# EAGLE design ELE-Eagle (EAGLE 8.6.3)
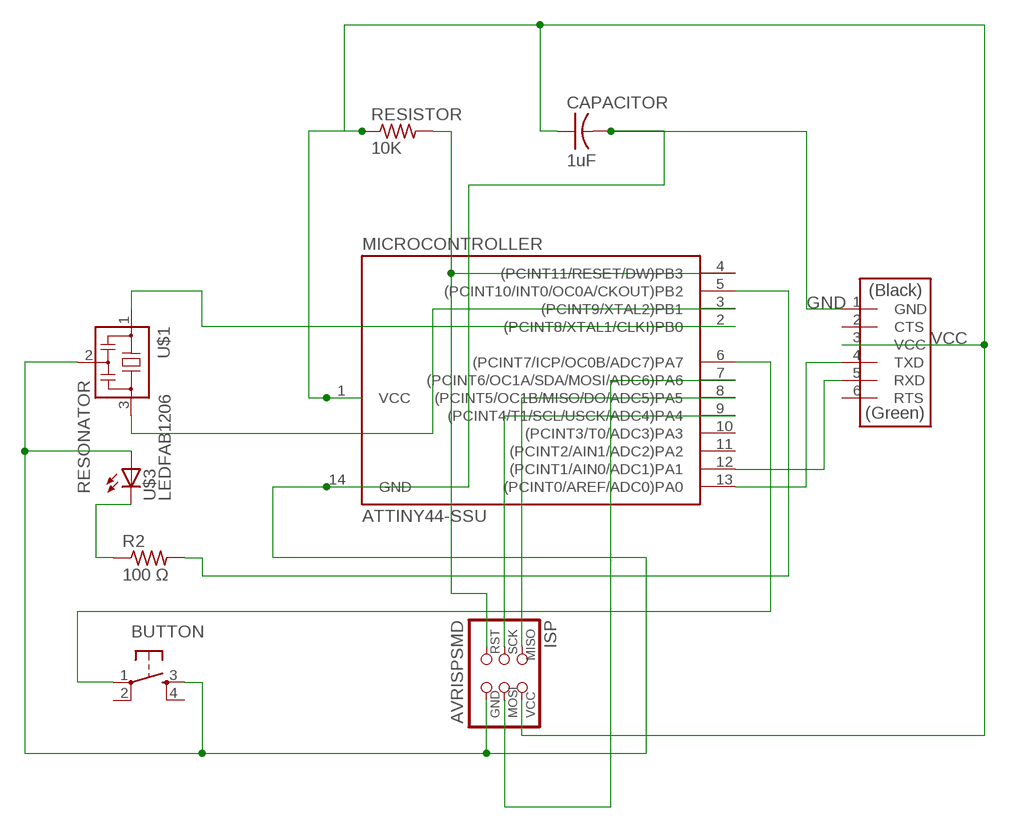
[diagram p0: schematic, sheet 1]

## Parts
BUTTON  6MM_SWITCH6MM_SWITCH  [6MM_SWITCH]
CAPACITOR  1uF  CAP-US1206FAB  [C1206FAB]
ISP  AVRISPSMD  [2X03SMD]
MICROCONTROLLER  ATTINY44-SSU  [SOIC14]
R2  100 Ω  RES-US1206FAB  [R1206FAB]
RESISTOR  10K  RES-US1206FAB  [R1206FAB]
U$1  RESONATOR  [EFOBM]
U$2  FTDI-SMD-HEADER  [1X06SMD]
U$3  LEDFAB1206  [LED1206FAB]

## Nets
GND: BUTTON.3(S) CAPACITOR.2 ISP.6(GND) MICROCONTROLLER.14(GND) U$1.2 U$2.1(GND) U$3.1(A)
N$1: BUTTON.1(P) MICROCONTROLLER.6((PCINT7/ICP/OC0B/ADC7)PA7)
N$2: ISP.4(MOSI) MICROCONTROLLER.7((PCINT6/OC1A/SDA/MOSI/ADC6)PA6)
N$4: MICROCONTROLLER.2((PCINT8/XTAL1/CLKI)PB0) U$1.1
N$5: MICROCONTROLLER.3((PCINT9/XTAL2)PB1) U$1.3
N$8: MICROCONTROLLER.13((PCINT0/AREF/ADC0)PA0) U$2.4(TXD)
N$9: MICROCONTROLLER.12((PCINT1/AIN0/ADC1)PA1) U$2.5(RXD)
N$10: ISP.5(RST) MICROCONTROLLER.4((PCINT11/RESET/DW)PB3) RESISTOR.2
N$11: ISP.3(SCK) MICROCONTROLLER.9((PCINT4/T1/SCL/USCK/ADC4)PA4)
N$12: ISP.1(MISO) MICROCONTROLLER.8((PCINT5/OC1B/MISO/DO/ADC5)PA5)
N$13: MICROCONTROLLER.5((PCINT10/INT0/OC0A/CKOUT)PB2) R2.2
N$14: R2.1 U$3.2(C)
VCC: CAPACITOR.1 ISP.2(VCC) MICROCONTROLLER.1(VCC) RESISTOR.1 U$2.3(VCC)
Unconnected: BUTTON.2(P1) BUTTON.4(S1) MICROCONTROLLER.10((PCINT3/T0/ADC3)PA3) MICROCONTROLLER.11((PCINT2/AIN1/ADC2)PA2) U$2.2(CTS) U$2.6(RTS)

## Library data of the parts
BUTTON = fab:6MM_SWITCH: OMRON SWITCH
CAPACITOR = fab:CAP-US
ISP = fab:AVRISP
MICROCONTROLLER = fab:ATTINY44
R2 RESISTOR = fab:RES-US: Resistor (US Symbol)
U$1 = fab:RESONATOR
U$2 = fab:FTDI-SMD-HEADER
U$3 = fab:LED: LED

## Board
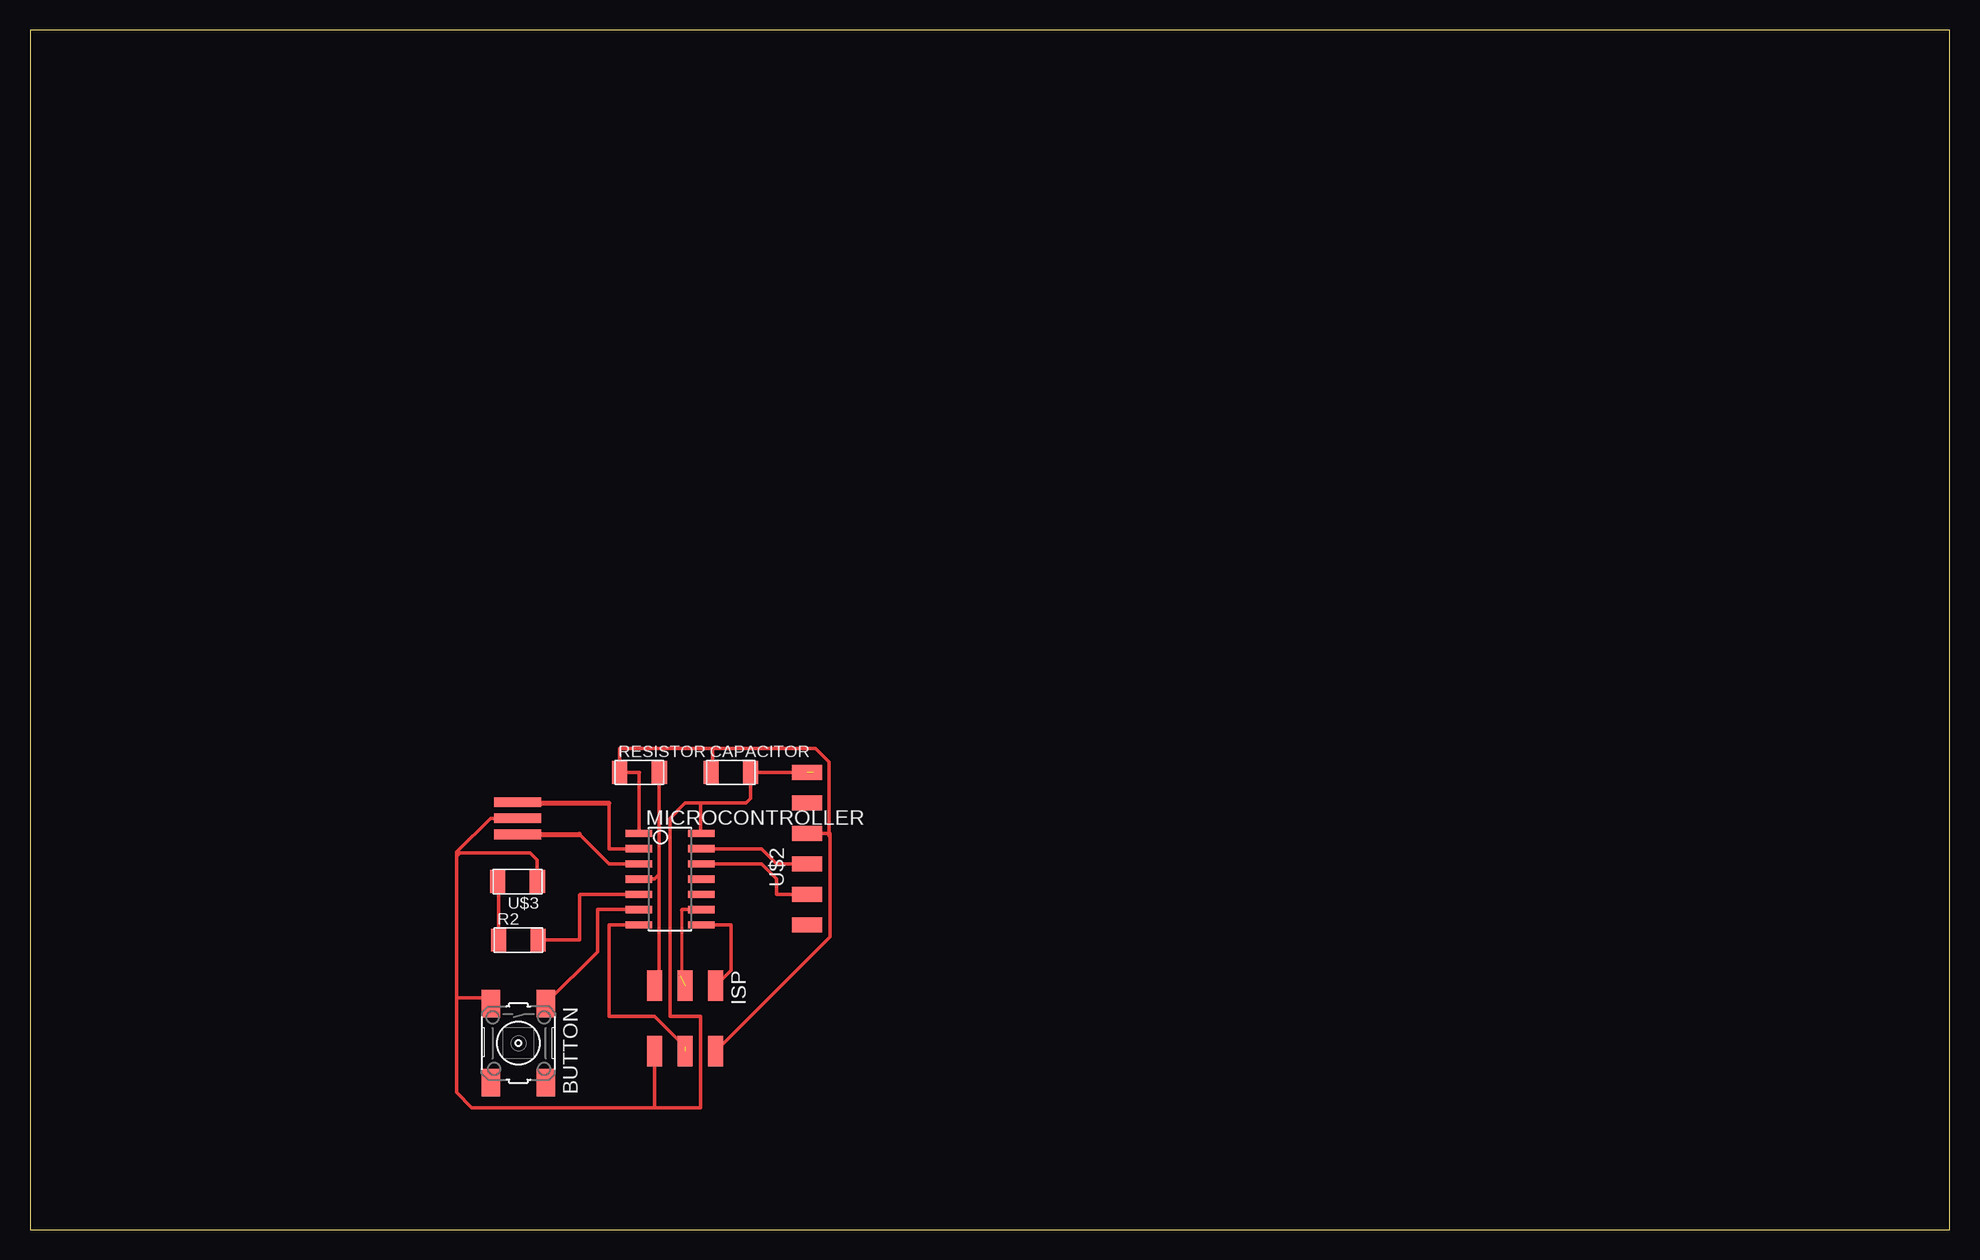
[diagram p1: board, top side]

Size 160 x 100 mm. Coordinates in mm from the lower left corner, seen from the top.
Outline: 0,0 160,0 160,100 0,100 0,0
Copper layers (1*16): Top 0.035mm / dielectric 1.5mm / Bottom 0.035mm
Design rules "default *": minimum track width 12mil, minimum drill 24mm, track to track 16mil, track to pad 16mil, pad to pad 16mil, via to via 16mil, smd to smd 6mil, copper to edge 40mil, drill to drill 6mil, minimum pad ring 10mil, minimum via ring 8mil, stop-mask expansion 4mil, vias tented up to drill 0mil, thermal gap 10mil

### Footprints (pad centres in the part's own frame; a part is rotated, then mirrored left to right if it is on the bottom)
6MM_SWITCH = smd 2.286 x 1.524: 1 -3.302,2.286; 2 3.302,2.286; 3 -3.302,-2.286; 4 3.302,-2.286
C1206FAB = smd 1.27 x 1.905: 1 -1.651,0; 2 1.651,0
2X03SMD = smd 2.54 x 1.27: 1 -2.54,2.54; 2 2.92,2.54; 3 -2.54,0; 4 2.92,0; 5 -2.54,-2.54; 6 2.92,-2.54
SOIC14 = smd 0.61 x 2.21: 1 -3.81,-2.603; 2 -2.54,-2.603; 3 -1.27,-2.603; 4 0,-2.603; 5 1.27,-2.603; 6 2.54,-2.603; 7 3.81,-2.603; 8 3.81,2.603; 9 2.54,2.603; 10 1.27,2.603; 11 0,2.603; 12 -1.27,2.603; 13 -2.54,2.603; 14 -3.81,2.603
R1206FAB = smd 1.27 x 1.905: 1 -1.651,0; 2 1.651,0
EFOBM = smd 0.8 x 3.9: 1 -1.35,0; 2 0,0; 3 1.35,0
1X06SMD = smd 2.54 x 1.27: 1 0,6.35; 2 0,3.81; 3 0,1.27; 4 0,-1.27; 5 0,-3.81; 6 0,-6.35
LED1206FAB = smd 1.27 x 1.905: 1 -1.651,0; 2 1.651,0

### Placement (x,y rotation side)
BUTTON  40.71,15.54 270 top
CAPACITOR  58.42,38.1 0 top
ISP  54.61,17.78 270 top
MICROCONTROLLER  53.34,29.21 270 top
R2  40.71,24.13 0 top
RESISTOR  50.8,38.1 0 top
U$1  40.64,34.29 270 top
U$2  64.77,31.75 0 top
U$3  40.64,29.01 180 top

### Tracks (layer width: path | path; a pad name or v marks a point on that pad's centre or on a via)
GND  (1 unrouted)
  Top 0.152: MICROCONTROLLER.14 55.88,33.08
  Top 0.305: U$1.2 38.39,34.29 35.56,31.46 35.56,31.1 | 35.56,31.1 35.56,19.3 | 35.56,19.3 35.56,11.43 36.83,10.16 52.07,10.16 | 52.07,10.16 ISP.6 | 52.07,10.16 55.88,10.16 55.88,17.78 53.34,17.78 53.34,34.29 54.61,35.56 55.88,35.56 | 55.88,35.56 59.69,35.56 60.07,35.94 CAPACITOR.2 65.3,38.1 | 55.88,33.08 55.88,35.56 | BUTTON.3 37.97,19.3 35.56,19.3 | U$3.1 42.29,30.81 41.7,31.4 35.86,31.4 35.56,31.1
N$1
  Top 0.305: BUTTON.1 47.3,23.15 47.3,26.7 50.71,26.7 MICROCONTROLLER.6
N$2  (1 unrouted)
  Top 0.305: MICROCONTROLLER.7 48.26,25.4 48.26,17.78 52.07,17.78 54.61,15.24
N$4
  Top 0.152: U$1.1 40.72,35.56
  Top 0.305: 48.26,35.56 48.26,31.75 MICROCONTROLLER.2
  Top 0.406: 40.72,35.56 48.26,35.56
N$5
  Top 0.305: 45.8,32.94 48.26,30.48 MICROCONTROLLER.3
  Top 0.406: U$1.3 45.8,32.94
N$8
  Top 0.305: MICROCONTROLLER.13 60.96,31.75 62.23,30.48 U$2.4
N$9
  Top 0.305: MICROCONTROLLER.12 60.96,30.48 62.23,29.21 62.23,27.94 U$2.5
N$10
  Top 0.152: 52.45,20.7 ISP.5
  Top 0.305: RESISTOR.2 52.45,29.59 | 52.45,29.59 52.07,29.21 MICROCONTROLLER.4 | 52.45,29.59 52.45,20.7
N$11  (1 unrouted)
  Top 0.254: 54.3,26.6 54.3,21.3
  Top 0.305: MICROCONTROLLER.9 54.37,26.67 54.3,26.6 | 54.3,21.3 54.2,21.2
N$12
  Top 0.305: ISP.1 58.42,21.59 58.42,25.4 MICROCONTROLLER.8
N$13
  Top 0.305: R2.2 45.8,24.13 45.8,27.9 45.84,27.94 MICROCONTROLLER.5
N$14
  Top 0.305: R2.1 39.06,28.94 U$3.2
VCC
  Top 0.152: MICROCONTROLLER.1 50.77,33.05 50.8,33.08 | 50.8,38.1 50.77,38.07
  Top 0.305: U$2.3 66.7,33.02 66.7,32.7 | 50.8,38.1 RESISTOR.1 49.15,40.1 56.9,40.1 | 50.77,38.07 50.77,33.05 | ISP.2 66.7,24.41 66.7,32.7 | CAPACITOR.1 56.9,38.23 56.9,40.1 | 66.7,32.7 66.6,32.8 66.6,38.97 65.47,40.1 56.9,40.1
